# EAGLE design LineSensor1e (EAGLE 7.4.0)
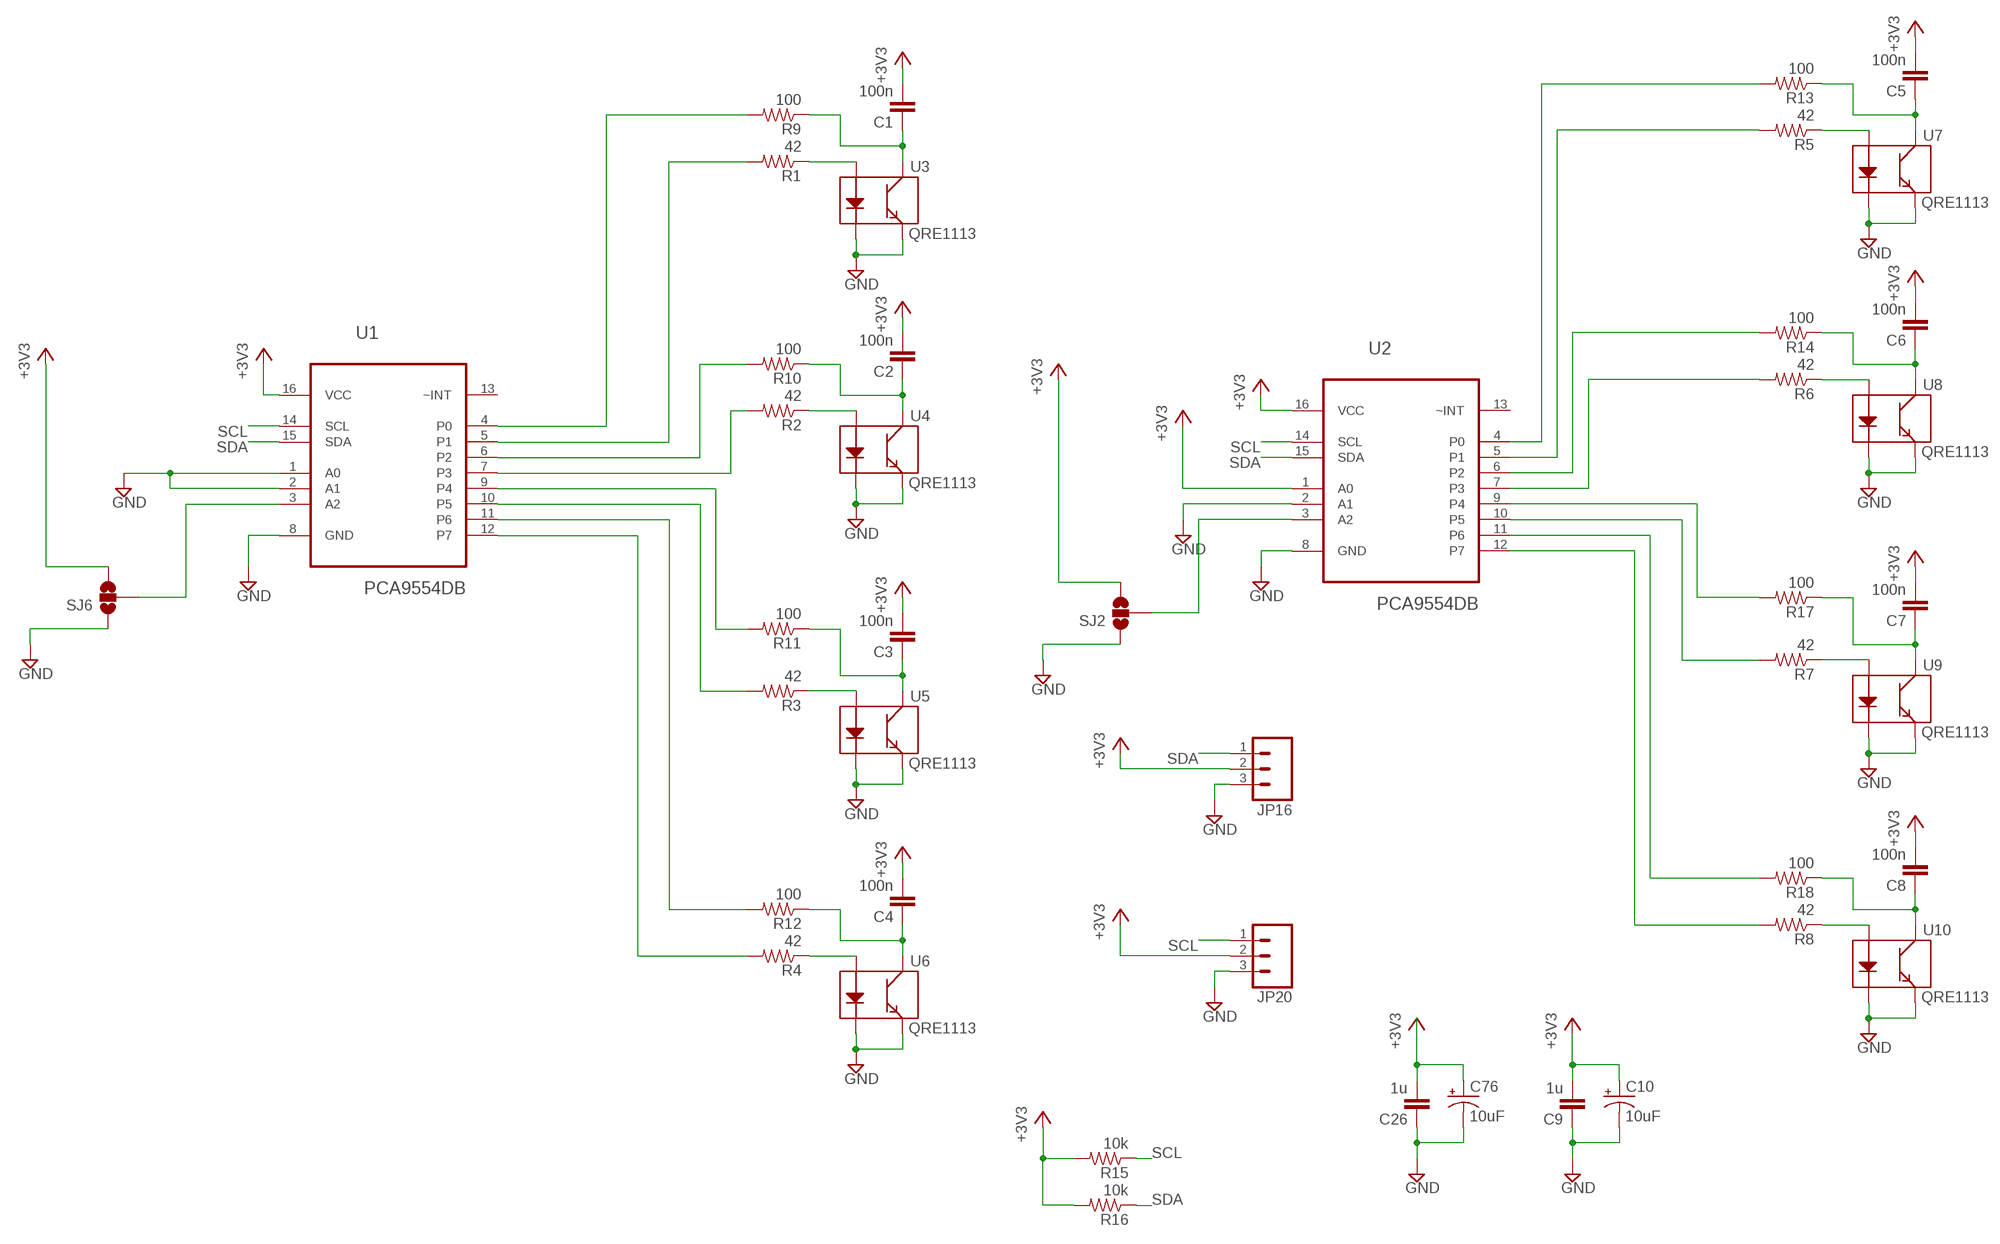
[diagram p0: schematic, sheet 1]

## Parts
C1  100n  C-EUC0805  [C0805]
C2  100n  C-EUC0805  [C0805]
C3  100n  C-EUC0805  [C0805]
C4  100n  C-EUC0805  [C0805]
C5  100n  C-EUC0805  [C0805]
C6  100n  C-EUC0805  [C0805]
C7  100n  C-EUC0805  [C0805]
C8  100n  C-EUC0805  [C0805]
C9  1u  C-EUC0805  [C0805]
C10  10uF  10UF-16V-10%(TANT)  [EIA3216]
C26  1u  C-EUC0805  [C0805]
C76  10uF  10UF-16V-10%(TANT)  [EIA3216]
JP16  M03PTH  [1X03]
JP20  M03PTH  [1X03]
R1  42  R-US_M0805  [M0805]
R2  42  R-US_M0805  [M0805]
R3  42  R-US_M0805  [M0805]
R4  42  R-US_M0805  [M0805]
R5  42  R-US_M0805  [M0805]
R6  42  R-US_M0805  [M0805]
R7  42  R-US_M0805  [M0805]
R8  42  R-US_M0805  [M0805]
R9  100  R-US_M0805  [M0805]
R10  100  R-US_M0805  [M0805]
R11  100  R-US_M0805  [M0805]
R12  100  R-US_M0805  [M0805]
R13  100  R-US_M0805  [M0805]
R14  100  R-US_M0805  [M0805]
R15  10k  R-US_M0805  [M0805]
R16  10k  R-US_M0805  [M0805]
R17  100  R-US_M0805  [M0805]
R18  100  R-US_M0805  [M0805]
SJ2  SOLDERJUMPER_2WAYPASTE1&2  [SJ_3_PASTE1&2]
SJ6  SOLDERJUMPER_2WAYPASTE1&2  [SJ_3_PASTE1&2]
U1  PCA9554DB  [SOP65P780X200-16N]
U2  PCA9554DB  [SOP65P780X200-16N]
U3  QRE1113  [QRE1113]
U4  QRE1113  [QRE1113]
U5  QRE1113  [QRE1113]
U6  QRE1113  [QRE1113]
U7  QRE1113  [QRE1113]
U8  QRE1113  [QRE1113]
U9  QRE1113  [QRE1113]
U10  QRE1113  [QRE1113]

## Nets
+3V3: C1.2 C2.2 C3.2 C4.2 C5.2 C6.2 C7.2 C8.2 C9.2 C10.A(+) C26.2 C76.A(+) JP16.2 JP20.2 R15.2 R16.2 SJ2.3 SJ6.3 U1.16(VCC) U2.1(A0) U2.16(VCC)
GND: C9.1 C10.C(-) C26.1 C76.C(-) JP16.3 JP20.3 SJ2.1 SJ6.1 U1.1(A0) U1.2(A1) U1.8(GND) U2.2(A1) U2.8(GND) U3.2(K) U3.4(E) U4.2(K) U4.4(E) U5.2(K) U5.4(E) U6.2(K) U6.4(E) U7.2(K) U7.4(E) U8.2(K) U8.4(E) U9.2(K) U9.4(E) U10.2(K) U10.4(E)
N$1: C1.1 R9.1 U3.3(C)
N$2: R1.1 U3.1(A)
N$3: R9.2 U1.4(P0)
N$4: R2.1 U4.1(A)
N$5: R3.1 U5.1(A)
N$6: C2.1 R10.1 U4.3(C)
N$7: R4.1 U6.1(A)
N$8: C3.1 R11.1 U5.3(C)
N$9: R5.1 U7.1(A)
N$10: C4.1 R12.1 U6.3(C)
N$11: R6.1 U8.1(A)
N$12: R1.2 U1.5(P1)
N$13: R7.1 U9.1(A)
N$14: R10.2 U1.6(P2)
N$15: R8.1 U10.1(A)
N$16: R2.2 U1.7(P3)
N$17: C5.1 R13.1 U7.3(C)
N$18: R11.2 U1.9(P4)
N$19: R3.2 U1.10(P5)
N$20: R12.2 U1.11(P6)
N$21: R4.2 U1.12(P7)
N$22: C6.1 R14.1 U8.3(C)
N$23: C7.1 R17.1 U9.3(C)
N$24: C8.1 R18.1 U10.3(C)
N$25: R13.2 U2.4(P0)
N$26: R5.2 U2.5(P1)
N$27: R14.2 U2.6(P2)
N$28: R6.2 U2.7(P3)
N$29: R17.2 U2.9(P4)
N$30: R7.2 U2.10(P5)
N$31: R18.2 U2.11(P6)
N$32: R8.2 U2.12(P7)
N$35: SJ2.2 U2.3(A2)
N$38: SJ6.2 U1.3(A2)
SCL: JP20.1 R15.1 U1.14(SCL) U2.14(SCL)
SDA: JP16.1 R16.1 U1.15(SDA) U2.15(SDA)
Unconnected: U1.13(~INT) U2.13(~INT)

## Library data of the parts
C1-C9 C26 = rcl:C-EU: CAPACITOR, European symbol
C10 C76 = SparkFun-Capacitors:10UF-16V-10%(TANT): CAP-00811; PROD_ID: CAP-00811
JP16 JP20 = SparkFun-Connectors:M03: Header 3 Standard 3-pin 0.1" header. Use with straight break away headers (SKU : PRT-00116), right angle break away headers (PRT-00553), swiss pins (PRT-00743), machine pins (PRT-00117), and female headers (PRT-00115). Molex polarized connector foot print use with SKU : PRT-08232 with associated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
R1-R18 = resistor:R-US_: RESISTOR, American symbol
SJ2 SJ6 = SparkFun-Passives:SOLDERJUMPER_2WAY: Solder Jumper 2 way solder jumper
U1 U2 = Texas Instruments_By_element14_Batch_1:PCA9554DB: REMOTE 8-BIT I2C AND SMBus I/O EXPANDER WITH INTERRUPT OUTPUT AND CONFIGURATION REGISTERS; MPN: PCA9554DB; OC_FARNELL: 1564918; OC_NEWARK: 06M7571; PACKAGE: SSOP-16; SUPPLIER: TEXAS INSTRUMENTS
U3-U10 = SparkFun:QRE1113

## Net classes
1 power: width 0.254 mm

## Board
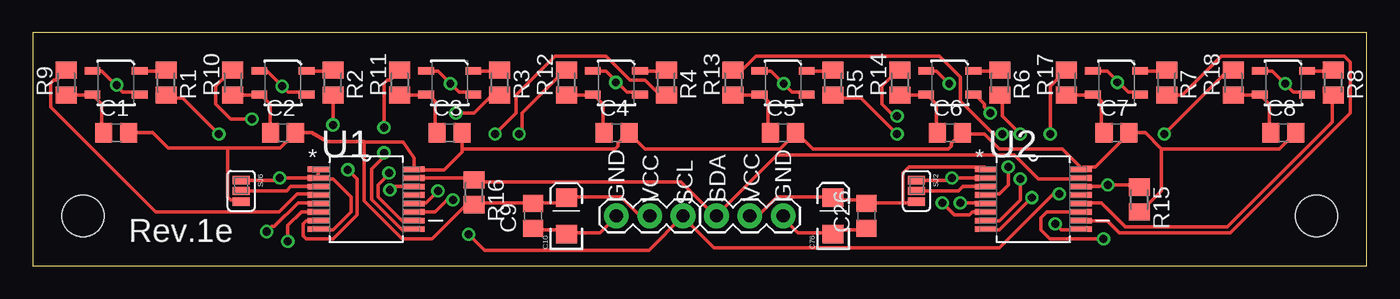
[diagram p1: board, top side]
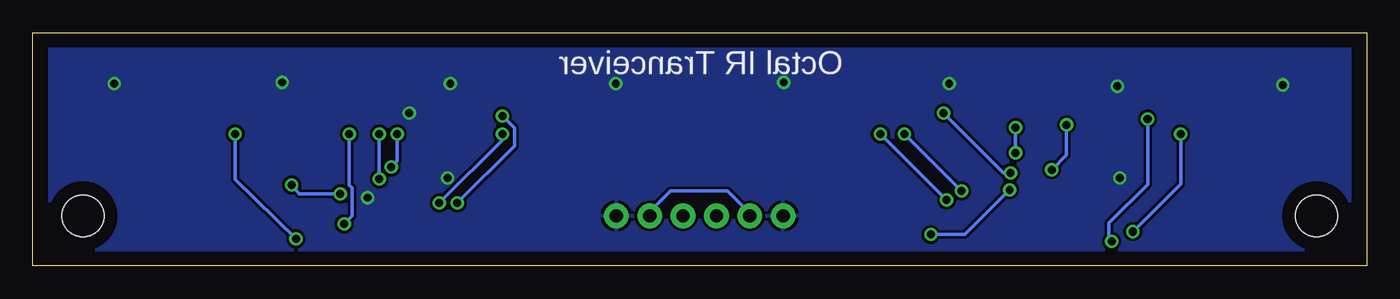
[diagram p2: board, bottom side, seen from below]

Size 101.6 x 17.78 mm. Coordinates in mm from the lower left corner, seen from the top.
Outline: 0,0 101.6,0 101.6,17.78 0,17.78 0,0
Copper layers (1*16): Top 0.035mm / dielectric 1.5mm / Bottom 0.035mm
Design rules "default": minimum track width 10mil, minimum drill 24mil, track to track 8mil, track to pad 8mil, pad to pad 8mil, via to via 8mil, smd to smd 8mil, copper to edge 40mil, drill to drill 8mil, minimum pad ring 10mil, minimum via ring 8mil, stop-mask expansion 4mil, vias tented up to drill 0mil, thermal gap 10mil
Holes 3.2 mm at 3.81,3.81 97.79,3.81

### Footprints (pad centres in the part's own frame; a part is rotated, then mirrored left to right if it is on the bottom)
C0805 = smd 1.3 x 1.5: 1 -0.95,0; 2 0.95,0
EIA3216 = smd 1.4 x 1.6: A 1.4,0; C -1.4,0
1X03 = drill 1.016 pad 1.88: 1 0,0; 2 2.54,0; 3 5.08,0
M0805 = smd 1.3 x 1.6: 1 -0.95,0; 2 0.95,0
SJ_3_PASTE1&2 = smd 0.635 x 1.27: 1 -0.813,0; 2 0,0; 3 0.813,0
SOP65P780X200-16N = smd 1.651 x 0.432: 1 -3.632,2.286; 2 -3.632,1.626; 3 -3.632,0.965; 4 -3.632,0.33; 5 -3.632,-0.33; 6 -3.632,-0.965; 7 -3.632,-1.626; 8 -3.632,-2.286; 9 3.632,-2.286; 10 3.632,-1.626; 11 3.632,-0.965; 12 3.632,-0.33; 13 3.632,0.33; 14 3.632,0.965; 15 3.632,1.626; 16 3.632,2.286
QRE1113 = smd 1.2 x 0.6: 1 -1.8,-0.9; 2 1.8,-0.9; 3 1.8,0.9; 4 -1.8,0.9

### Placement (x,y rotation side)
C1  6.35,10.16 0 top
C2  19.05,10.16 0 top
C3  31.75,10.16 0 top
C4  44.45,10.16 0 top
C5  57.15,10.16 0 top
C6  69.85,10.16 0 top
C7  82.55,10.16 0 top
C8  95.25,10.16 0 top
C9  38.1,3.81 90 top
C10  40.64,3.81 90 top
C26  63.5,3.81 90 top
C76  60.96,3.81 90 top
JP16  52.07,3.81 0 top
JP20  49.53,3.81 180 top
R1  10.16,13.97 270 top
R2  22.86,13.97 270 top
R3  35.56,13.97 270 top
R4  48.26,13.97 270 top
R5  60.96,13.97 270 top
R6  73.66,13.97 270 top
R7  86.36,13.97 270 top
R8  99.06,13.97 270 top
R9  2.54,13.97 90 top
R10  15.24,13.97 90 top
R11  27.94,13.97 90 top
R12  40.64,13.97 90 top
R13  53.34,13.97 90 top
R14  66.04,13.97 90 top
R15  84.29,5.05 270 top
R16  33.61,5.62 270 top
R17  78.74,13.97 90 top
R18  91.44,13.97 90 top
SJ2  67.31,5.71 270 top
SJ6  15.88,5.71 270 top
U1  25.4,5.08 0 top
U2  76.2,5.08 0 top
U3  6.35,13.97 180 top
U4  19.05,13.97 180 top
U5  31.75,13.97 180 top
U6  44.45,13.97 180 top
U7  57.15,13.97 180 top
U8  69.85,13.97 180 top
U9  82.55,13.97 180 top
U10  95.25,13.97 180 top

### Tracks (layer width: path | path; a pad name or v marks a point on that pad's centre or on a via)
+3V3
  Top 0.254: C1.2 9.14,10.16 10.3,9 14.86,9 | 14.86,9 18.84,9 C2.2 21.24,10.16 22.4,9.5 25.25,9.5 | 25.25,9.5 25.23,9.1 25.23,4.94 28.12,2.06 30.4,2.06 32.92,4.57 33.6,4.57 R16.2 33.83,4.8 37.95,4.8 C9.2 38.18,4.8 40.23,4.8 40.46,5.03 C10.A 40.69,5.26 44.81,5.26 46.18,3.89 46.86,3.89 JP20.2 | 85.97,8.93 84.74,10.16 C7.2 83.44,10.06 80.92,7.54 80.01,7.54 U2.16 79.78,7.54 78.41,8.91 73.61,8.91 72.47,10.06 70.87,10.06 C6.2 70.64,10.06 69.95,9.37 69.95,9.14 69.72,8.91 59.44,8.91 58.29,10.06 C5.2 58.06,10.06 56.92,8.91 46.63,8.91 45.49,10.06 C4.2 45.26,10.06 44.58,9.37 44.58,9.14 44.35,8.91 32.69,8.91 | 85.97,8.93 86,8.9 94.94,8.9 C8.2 | 66.29,4.8 63.55,4.8 C26.2 63.32,4.8 63.09,5.03 61.04,5.03 C76.A 60.81,5.26 56.69,5.26 55.32,3.89 54.63,3.89 JP16.2 | 66.29,4.8 67.21,4.8 SJ2.3 | 66.29,4.8 66.29,7.09 66.75,7.54 72.47,7.54 U2.1 | 14.86,9 14.86,5.26 15.09,5.03 15.77,5.03 SJ6.3 | R15.2 84.35,4.12 85.95,5.71 85.95,8.91 85.97,8.93 | 32.69,8.91 32.69,8.69 31.32,7.32 29.03,7.32 U1.16 29.03,8.23 28.22,9.44 25.25,9.44 25.25,9.5 | 32.69,8.91 32.69,10.06 C3.2
  Bottom 0.254: JP16.2 54.41,3.89 54.41,4.34 53.03,5.71 48.69,5.71 46.86,3.89 JP20.2
GND  (via drill 0.6, 0.61)
  Top 0.254: SJ6.1 18.63,6.53 v18.8,6.7 U1.2 | SJ2.1 69.83,6.53 v70,6.7 v70.01,6.71 U2.2 | C26.1 63.32,2.74 61.27,2.74 61.04,2.52 C76.C 60.81,2.52 58.29,2.52 57.15,3.66 JP16.3 | C9.1 38.18,2.74 40.23,2.74 40.46,2.52 C10.C 40.69,2.52 43.2,2.52 44.35,3.66 JP20.3 | U3.4 8,13.26 6.86,13.26 6.4,13.72 v6.4,13.8 6.17,13.95 5.26,14.86 4.57,14.86 U3.2 | U4.2 17.37,14.86 17.83,14.86 18.97,13.72 v19,13.7 19.2,13.49 19.43,13.26 20.8,13.26 U4.4 | U5.2 30.18,14.86 30.86,14.86 31.77,13.95 v31.8,13.9 32,13.72 32.46,13.26 33.38,13.26 U5.4 | U6.2 42.75,14.86 43.66,14.86 44.35,14.17 v44.4,14 44.58,13.95 45.26,13.26 46.18,13.26 U6.4 | U7.2 55.55,14.86 56.24,14.86 57.15,13.95 v57.2,13.9 57.38,13.72 57.84,13.26 58.75,13.26 U7.4 | U8.2 68.12,14.86 68.81,14.86 69.72,13.95 v69.8,13.9 | v72.92,11.66 72.47,12.12 72.47,12.34 71.78,13.03 U8.4 | U9.2 80.92,14.86 81.84,14.86 82.53,14.17 v82.6,14 82.75,13.95 83.44,13.26 84.12,13.26 U9.4 | U10.2 93.5,14.86 94.41,14.86 95.33,13.95 v95.4,13.9 95.56,13.72 96.01,13.26 96.93,13.26 U10.4 | U1.1 21.72,7.32 21.72,6.86 U1.2 | U2.8 72.69,2.74 73.61,2.74 75.89,5.03 v76.1,5.2 | U1.8 21.95,2.74 22.86,2.74 24.23,4.12 24.23,5.26 22.86,6.63 21.95,6.63 U1.2
  pour Bottom: 1.27,16.51 100.33,16.51 100.33,1.27 1.27,1.27
N$1
  Top 0.254: R9.1 2.74,13.03 4.34,13.03 U3.3 4.57,13.03 5.26,12.34 5.26,10.29 C1.1
N$2
  Top 0.254: U3.1 8.23,14.86 10.06,14.86 R1.1
N$3
  Top 0.254: R9.2 2.52,14.86 1.83,14.17 1.6,14.17 1.37,13.95 1.37,12.12 9.37,4.12 18.75,4.12 20.12,5.49 21.72,5.49 U1.4
N$4
  Top 0.254: U4.1 21.03,14.86 22.86,14.86 R2.1
N$5
  Top 0.254: U5.1 33.6,14.86 35.43,14.86 R3.1
N$6
  Top 0.254: R10.1 15.32,13.03 17.14,13.03 U4.3 17.37,13.03 18.06,12.34 18.06,10.29 C2.1
N$7
  Top 0.254: U6.1 46.41,14.86 48.23,14.86 R4.1
N$8
  Top 0.254: R11.1 28.12,13.03 29.95,13.03 U5.3 30.18,13.03 30.63,12.57 30.63,10.29 C3.1
N$9
  Top 0.254: U7.1 58.98,14.86 60.81,14.86 R5.1
N$10
  Top 0.254: R12.1 40.69,13.03 42.52,13.03 U6.3 42.75,13.03 43.43,12.34 43.43,10.29 C4.1
N$11
  Top 0.254: U8.1 71.78,14.86 73.61,14.86 R6.1
N$12  (via drill 0.61)
  Top 0.254: v14.17,10.06 11.43,12.8 10.29,12.8 R1.2 | U1.5 21.72,4.8 20.2,4.8 18.4,3 18.2,3 v17.82,2.62
  Bottom 0.254: v17.82,2.62 14.17,6.26 v14.17,10.06
N$13
  Top 0.254: U9.1 86.18,14.86 R7.1
N$14  (via drill 0.61)
  Top 0.254: v16.69,11.2 15.09,11.2 13.95,12.34 13.95,13.72 15.09,14.86 R10.2 | U1.6 20.46,4.12 19.42,3.07 v19.42,1.87
  Bottom 0.254: v16.69,11.2 16.69,6.21 19.62,3.28 19.62,2.08 v19.42,1.87
N$15
  Top 0.254: U10.1 97.16,14.86 98.98,14.86 R8.1
N$16  (via drill 0.61)
  Top 0.254: v22.86,10.76 R2.2 | 21.95,3.43 U1.7 21.72,3.43 20.8,3.43 20.57,3.2 20.57,2.29 20.8,2.06 22.86,2.06 24.69,3.89 24.69,6.63 v23.99,7.33
  Bottom 0.254: v22.86,10.76 22.86,8.46 v23.99,7.33
N$17
  Top 0.254: R13.1 53.49,13.03 55.32,13.03 U7.3 55.55,13.03 56.01,12.57 56.01,10.29 C5.1
N$18  (via drill 0.61)
  Top 0.254: v26.75,10.56 26.75,13.95 26.98,14.17 27.2,14.17 27.89,14.86 R11.2 | U1.9 29.03,2.74 28.12,2.74 25.8,5.06 25.8,7.4 26.63,8.23 v26.75,8.63
  Bottom 0.254: v26.75,8.63 v26.75,10.56
N$19  (via drill 0.61)
  Top 0.254: U1.10 29.03,3.43 28.12,3.43 26.3,5.25 26.3,6.18 27.2,7.09 v27.13,7.09 | v32.23,11.66 33.6,11.66 34.75,12.8 35.43,12.8 R3.2
  Bottom 0.254: v32.23,11.66 27.66,7.09 v27.13,7.09
N$20  (via drill 0.61)
  Top 0.254: v37.03,10.06 37.26,10.29 37.26,11.66 40.46,14.86 R12.2 | v32,5.03 31.55,5.03 30.63,4.12 U1.11
  Bottom 0.254: v32,5.03 v37.03,10.06
N$21  (via drill 0.61)
  Top 0.254: v35.2,10.06 36.8,11.66 36.8,13.03 39.78,16 43.66,16 45.49,14.17 46.63,14.17 47.78,13.03 48.23,13.03 R4.2 | v30.86,5.71 29.95,4.8 29.03,4.8 U1.12
  Bottom 0.254: v30.86,5.71 v35.2,10.06
N$22
  Top 0.254: R14.1 66.06,13.03 67.89,13.03 U8.3 68.12,13.03 68.81,12.34 68.81,10.29 C6.1
N$23
  Top 0.254: R17.1 78.87,13.03 80.7,13.03 U9.3 80.92,13.03 81.38,12.57 81.38,10.29 C7.1
N$24
  Top 0.254: R18.1 93.27,13.03 U10.3 93.5,13.03 94.18,12.34 94.18,10.29 C8.1
N$25  (via drill 0.61)
  Top 0.254: v73.84,10.06 73.15,10.06 70.64,12.57 70.64,14.4 69.04,16 55.09,16 54.18,15.09 53.49,15.09 R13.2 | v74.3,7.54 74.3,6.17 73.61,5.49 72.69,5.49 U2.4
  Bottom 0.254: v73.84,10.06 73.84,8 v74.3,7.54
N$26  (via drill 0.61)
  Top 0.254: v65.84,10.06 63.09,12.8 61.04,12.8 R5.2 | v70.64,4.8 72.47,4.8 U2.5
  Bottom 0.254: v65.84,10.06 65.84,9.6 v70.64,4.8
N$27  (via drill 0.61)
  Top 0.254: v65.84,11.43 65.61,11.43 64.69,12.34 64.69,13.72 65.84,14.86 R14.2 | v69.27,4.8 70.18,3.89 71.32,3.89 71.55,4.12 U2.6
  Bottom 0.254: v65.84,11.43 64.92,10.52 64.92,9.14 v69.27,4.8
N$28  (via drill 0.61)
  Top 0.254: v75.21,10.06 73.84,11.43 73.84,12.8 R6.2 | v75.21,6.63 75.21,5.03 73.61,3.43 72.69,3.43 U2.7
  Bottom 0.254: v75.21,6.63 v75.21,10.06
N$29  (via drill 0.61)
  Top 0.254: v77.5,10.06 77.5,13.72 78.64,14.86 R17.2 | v77.88,3.2 78.34,2.74 79.78,2.74 U2.9
  Bottom 0.254: v77.5,10.06 77.5,6.17 77.27,5.94 77.27,3.81 v77.88,3.2
N$30
  Top 0.254: R7.2 86.41,13.03 87.55,13.03 90.53,16 99.9,16 100.36,15.54 100.36,11.66 91.21,2.52 82.77,2.52 81.85,3.43 80.01,3.43 U2.10
N$31  (via drill 0.61)
  Top 0.254: v86.18,10.06 90.98,14.86 91.44,14.86 R18.2 | v81.55,2.06 77.45,2.06 76.77,2.74 76.77,3.66 77.22,4.12 U2.11
  Bottom 0.254: v86.18,10.06 86.18,6.59 v81.55,2.06
N$32
  Top 0.254: R8.2 98.98,12.8 98.98,10.97 90.98,2.97 83.22,2.97 81.4,4.8 80.01,4.8 U2.12
N$35
  Top 0.254: SJ2.2 70.52,5.71 70.84,6.04 U2.3
N$38
  Top 0.254: SJ6.2 19.32,5.71 19.64,6.04 U1.3
SCL  (via drill 0.6, 0.61)
  Top 0.254: v78.18,5.49 77.72,5.49 73.61,1.37 51.89,1.37 49.61,3.66 JP20.1 46.92,1.2 34.4,1.2 v33.2,2.4 | R15.1 84.12,6.17 v81.88,6.17 81.25,6.04 U2.14 | U1.14 27.45,6.04 v27.2,5.8
  Bottom 0.254: v81.88,6.17 81.3,5.49 v78.18,5.49 | v27.2,5.8 30.6,2.4 v33.2,2.4
SDA
  Top 0.254: U1.15 33.47,6.71 R16.1 33.83,6.4 49.38,6.4 51.89,3.89 JP16.1 52.12,3.89 56.69,8.46 74.75,8.46 76.58,6.63 79.78,6.63 U2.15

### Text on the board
tPlace: GND | VCC | GND | VCC | SCL | SDA | Rev.1e
bPlace: Octal IR Tranceiver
